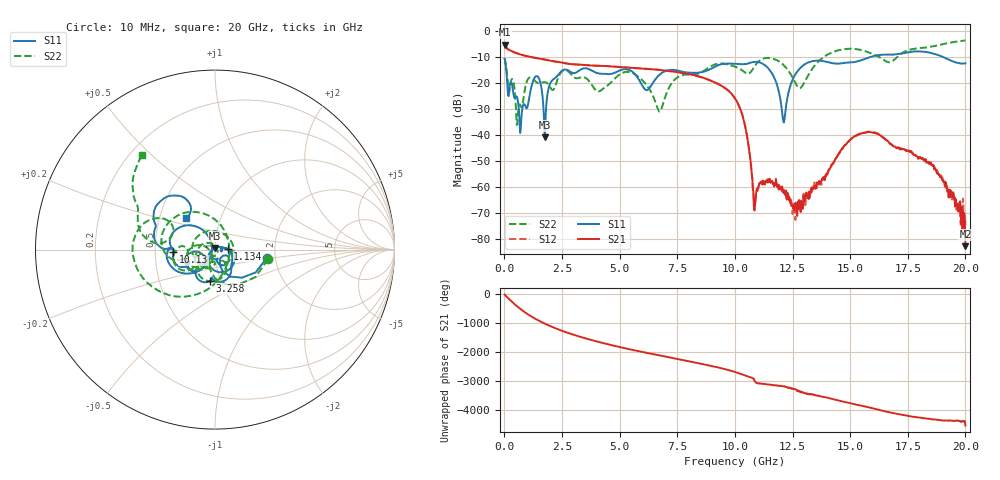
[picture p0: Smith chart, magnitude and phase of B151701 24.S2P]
!  2-Port S-parameters saved by WinCal
! VAR MeasName=S-Parameters (CALIBRATED_DATA) read from VNA (N5244A)
! VAR MeasDate=2015-12-24 19:10:56
! VAR NAME=B151701 24
! VAR FILENAME=B151701 24.S2P
! VAR DATE=2015-12-24 19:10:56
! VAR PHYS_PORTS=1,3
# Hz S DB R 50
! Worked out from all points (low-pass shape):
!   801 points, 10 MHz to 20 GHz, reference 50 ohm
!   highest |S21| = -5.16 dB at 10 MHz (marker M1); lowest = -82.8 dB at 20 GHz (marker M2)
!   |S21| within 3 dB of the highest: start of sweep to 430 MHz
!   lowest |S11| = -40.9 dB at 1.759 GHz (marker M3), VSWR 1.02, Z = 50.1 + j0.904 ohm
!   |S11| at or under -10 dB: start of sweep to 15.86 GHz; 19.04 GHz to end of sweep
!   |S22| runs from -36.1 to -3.6 dB; largest |S21 - S12| = 0.00095
!   S11 on the Smith chart (normalised r, x): 10 MHz: 1.80, -0.18; 1.134 GHz: 1.15, +0.01; 3.258 GHz: 0.89, -0.32; 10.13 GHz: 0.62, -0.02; 20 GHz: 0.68, +0.25
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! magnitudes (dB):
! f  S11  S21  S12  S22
! 10 MHz  -10.7  -5.2  -5.2  -10.5
! 609.7 MHz  -28.4  -8.7  -8.7  -29.9
! 1.134 GHz  -22.9  -9.9  -9.9  -17.8
! 1.459 GHz  -17.6  -10.5  -10.4  -20.0
! 1.759 GHz  -40.9  -10.9  -10.9  -19.6
! 2.084 GHz  -18.8  -11.5  -11.5  -22.7
! 3.258 GHz  -15.1  -12.9  -12.9  -17.9
! 3.358 GHz  -14.6  -13.0  -13.0  -17.7
! 5.532 GHz  -15.5  -14.2  -14.1  -16.0
! 6.682 GHz  -17.2  -14.9  -14.9  -30.4
! 7.556 GHz  -15.2  -15.9  -15.8  -17.6
! 10.01 GHz  -12.6  -25.9  -25.8  -13.7
! 10.13 GHz  -12.6  -27.8  -27.8  -14.1
! 10.88 GHz  -11.8  -66.5  -66.9  -13.2
! 11.63 GHz  -16.6  -57.7  -59.2  -10.5
! 12.13 GHz  -35.2  -62.5  -62.3  -13.2
! 12.8 GHz  -14.5  -66.9  -66.9  -21.9
! 13.35 GHz  -11.6  -60.4  -61.8  -14.5
! 15.18 GHz  -11.9  -40.5  -40.8  -6.8
! 16.68 GHz  -9.0  -42.8  -42.7  -12.0
! 18.53 GHz  -8.4  -51.4  -51.6  -5.9
! 20 GHz  -12.4  -82.8  -72.9  -3.6
